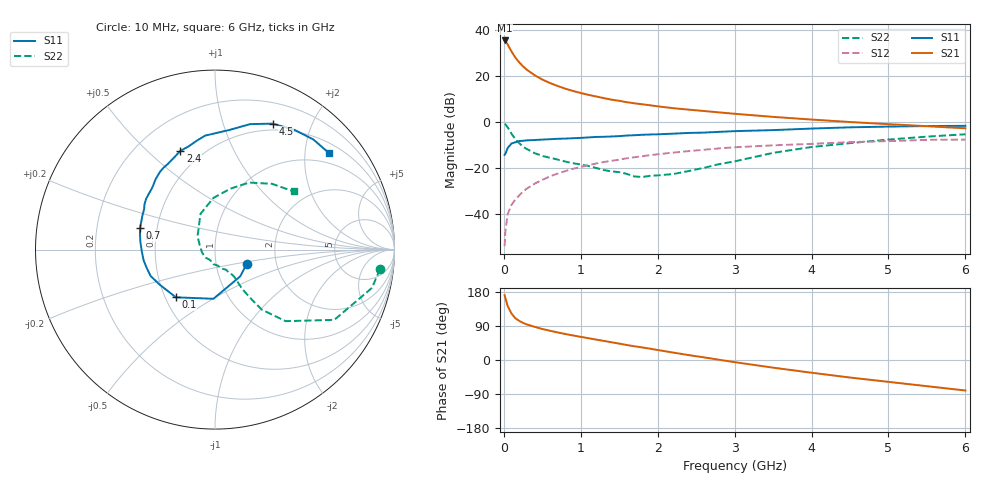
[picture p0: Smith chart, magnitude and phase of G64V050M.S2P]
! SIEMENS Small Signal Semiconductors
! BFG193
! Si NPN RF Bipolar Junction Transistor in SOT223
! VCE = 4 V  IC = 50 mA
! Common Emitter S-Parameters:  August  1996
# GHz  S  MA  R  50
!  f  S11  S21  S12  S22
! GHz  MAG  ANG  MAG  ANG  MAG  ANG  MAG  ANG
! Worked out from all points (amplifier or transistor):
!   36 points, 10 MHz to 6 GHz, reference 50 ohm
!   highest |S21| = 35.6 dB at 10 MHz (marker M1)
!   |S21| within 3 dB of that: start of sweep to 70.2 MHz
!   unconditionally stable (mu >= 1): 432.5 MHz to 2.35 GHz
!   at 250 MHz: K = 0.92, MSG = 27.2 dB, |S12| = -30.2 dB
!   at 1.4 GHz: K = 1.05, MAG = 12.0 dB, |S12| = -16.8 dB
!   at 6 GHz: K = 0.90, MSG = 2.5 dB, |S12| = -7.6 dB
!   S11 on the Smith chart (normalised r, x): 10 MHz: 1.40, -0.24; 100 MHz: 0.57, -0.34; 700 MHz: 0.40, +0.12; 2.4 GHz: 0.38, +0.64; 4.5 GHz: 0.42, +1.47; 6 GHz: 0.73, +2.55
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0.01  0.194 -24.8  60.03 171.0  0.002 87.7  0.9257 -6.7
0.02  0.2049 -46.8  57.73 163.3  0.0042 78.2  0.9003 -13.7
0.05  0.2742 -91.8  48.85 142.4  0.01 71.6  0.7714 -30.5
0.1  0.3439 -129.4  34.61 122.5  0.016 67.6  0.56 -45.4
0.15  0.3654 -147.9  25.42 110.1  0.0207 66.6  0.4247 -52.0
0.2  0.3877 -157.7  20.03 103.2  0.0255 68.0  0.3476 -53.6
0.25  0.394 -164.9  16.33 97.8  0.0309 68.7  0.2915 -54.8
0.3  0.402 -171.3  13.82 93.7  0.0359 69.4  0.2593 -55.3
0.4  0.4083 -178.8  10.53 87.6  0.0458 69.2  0.212 -55.0
0.5  0.4181 174.0  8.455 81.8  0.0556 68.3  0.1842 -54.7
0.6  0.4255 169.1  7.107 77.2  0.066 67.7  0.168 -55.8
0.7  0.4346 164.2  6.122 72.7  0.0762 66.5  0.1532 -57.9
0.9  0.4469 154.8  4.774 64.7  0.0965 62.6  0.1276 -61.3
1.1  0.4656 147.7  3.929 57.5  0.1158 59.1  0.1113 -71.1
1.3  0.4808 140.8  3.337 50.3  0.1358 55.2  0.0906 -80.0
1.6  0.5119 130.5  2.718 39.5  0.1637 48.3  0.0747 -103.5
2.2  0.5618 113.8  2.017 19.7  0.2174 34.7  0.0742 -168.6
2.4  0.583 109.4  1.874 13.0  0.2338 30.4  0.0862 166.8
3.5  0.6716 83.1  1.303 -20.2  0.3131 3.4  0.2149 112.1
4.5  0.7719 65.4  1.007 -46.3  0.3676 -16.6  0.35 75.9
5.5  0.8226 48.2  0.817 -69.1  0.4124 -40.0  0.4846 49.2
6  0.8324 40.2  0.736 -80.5  0.4181 -53.3  0.5448 36.5
